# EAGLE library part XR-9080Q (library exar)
DATA SYNCHRONIZER/RLL ENDEC
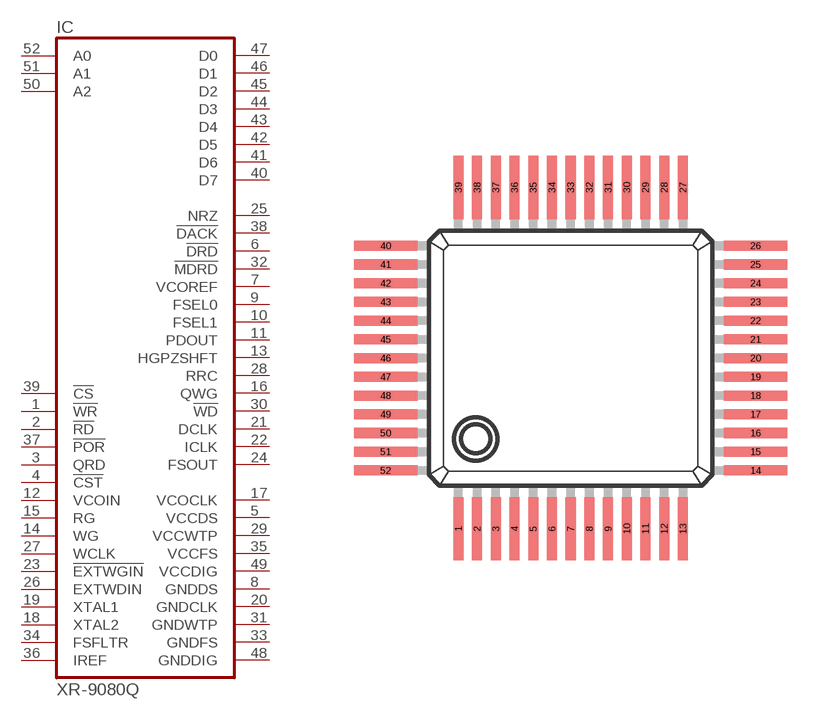
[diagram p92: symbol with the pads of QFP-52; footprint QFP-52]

Designator prefix IC

## XR-9080Q (OC_FARNELL: unknown; OC_NEWARK: unknown)  [QFP-52]
1  !WR  in
2  !RD  in
3  QRD  in
4  !CST  in
5  VCCDS  pwr
6  !DRD  out
7  VCOREF  out
8  GNDDS  pwr
9  FSEL0  out
10  FSEL1  out
11  PDOUT  out
12  VCOIN  in
13  HGPZSHFT  out
14  WG  in
15  RG  in
16  QWG  out
17  VCOCLK  out
18  XTAL2  in
19  XTAL1  in
20  GNDCLK  pwr
21  DCLK  out
22  ICLK  out
23  !EXTWGIN  in
24  FSOUT  out
25  NRZ
26  EXTWDIN  in
27  WCLK  in
28  RRC  out
29  VCCWTP  pwr
30  !WD  out
31  GNDWTP  pwr
32  !MDRD  out
33  GNDFS  pwr
34  FSFLTR  in
35  VCCFS  pwr
36  IREF  in
37  !POR  in
38  !DACK  out
39  !CS  in
40  D7
41  D6
42  D5
43  D4
44  D3
45  D2
46  D1
47  D0
48  GNDDIG  pwr
49  VCCDIG  pwr
50  A2  in
51  A1  in
52  A0  in

## Footprint QFP-52 (pad centres in mm)
Quad Flat Package
smd 0.35 x 2.2: 1 -3.575,-6.25; 2 -2.925,-6.25; 3 -2.275,-6.25; 4 -1.625,-6.25; 5 -0.975,-6.25; 6 -0.325,-6.25; 7 0.325,-6.25; 8 0.975,-6.25; 9 1.625,-6.25; 10 2.275,-6.25; 11 2.925,-6.25; 12 3.575,-6.25; 13 4.225,-6.25; 27 4.225,5.6; 28 3.575,5.6; 29 2.925,5.6; 30 2.275,5.6; 31 1.625,5.6; 32 0.975,5.6; 33 0.325,5.6; 34 -0.325,5.6; 35 -0.975,5.6; 36 -1.625,5.6; 37 -2.275,5.6; 38 -2.925,5.6; 39 -3.575,5.6
smd 2.2 x 0.35: 14 6.75,-4.225; 15 6.75,-3.575; 16 6.75,-2.925; 17 6.75,-2.275; 18 6.75,-1.625; 19 6.75,-0.975; 20 6.75,-0.325; 21 6.75,0.325; 22 6.75,0.975; 23 6.75,1.625; 24 6.75,2.275; 25 6.75,2.925; 26 6.75,3.575; 40 -6.1,3.575; 41 -6.1,2.925; 42 -6.1,2.275; 43 -6.1,1.625; 44 -6.1,0.975; 45 -6.1,0.325; 46 -6.1,-0.325; 47 -6.1,-0.975; 48 -6.1,-1.625; 49 -6.1,-2.275; 50 -6.1,-2.925; 51 -6.1,-3.575; 52 -6.1,-4.225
